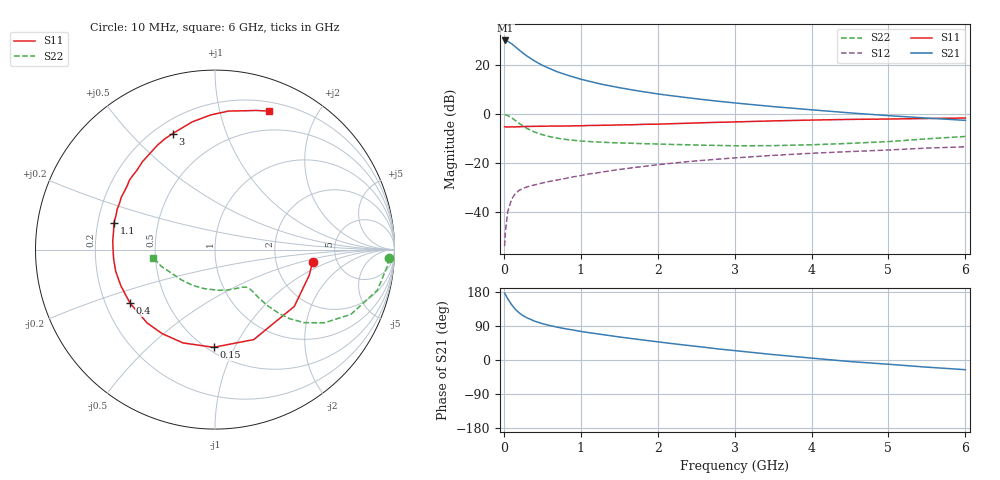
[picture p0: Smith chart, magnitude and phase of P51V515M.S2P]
! SIEMENS Small Signal Semiconductors
! BFP183
! Si NPN RF Bipolar Junction Transistor in SOT143
! VCE = 1.5 V  IC = 15 mA
! Common Emitter S-Parameters:  March  1996
# GHz  S  MA  R  50
!  f  S11  S21  S12  S22
! GHz  MAG  ANG  MAG  ANG  MAG  ANG  MAG  ANG
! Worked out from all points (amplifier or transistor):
!   36 points, 10 MHz to 6 GHz, reference 50 ohm
!   highest |S21| = 30.0 dB at 20 MHz (marker M1)
!   |S21| within 3 dB of that: start of sweep to 165.3 MHz
!   unconditionally stable (mu >= 1): 853.1 MHz to 5.693 GHz
!   at 250 MHz: K = 0.44, MSG = 27.6 dB, |S12| = -30.4 dB
!   at 1.4 GHz: K = 1.15, MAG = 14.9 dB, |S12| = -23.1 dB
!   at 6 GHz: K = 0.97, MSG = 5.4 dB, |S12| = -13.4 dB
!   S11 on the Smith chart (normalised r, x): 10 MHz: 3.29, -0.65; 150 MHz: 0.54, -0.83; 400 MHz: 0.30, -0.26; 1.1 GHz: 0.27, +0.12; 3 GHz: 0.27, +0.67; 6 GHz: 0.29, +1.42
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0.01  0.5485 -7.2  31.71 176.3  0.002 86.2  0.9715 -2.8
0.02  0.544 -15.3  31.73 172.9  0.0039 81.7  0.9635 -5.7
0.05  0.5436 -35.6  30.63 161.7  0.01 79.4  0.9328 -14.0
0.1  0.5458 -66.7  27.16 146.2  0.0182 64.0  0.8388 -25.5
0.15  0.5445 -90.8  23.52 133.7  0.0238 56.3  0.733 -33.8
0.2  0.5497 -108.9  20.23 124.3  0.0276 51.6  0.6425 -39.3
0.25  0.5531 -122.2  17.42 117.0  0.0302 47.8  0.5685 -42.7
0.3  0.5569 -132.7  15.29 111.4  0.0324 45.8  0.5082 -44.8
0.4  0.5596 -147.9  12.09 102.5  0.0357 45.1  0.4275 -46.9
0.5  0.5619 -159.0  9.865 96.0  0.039 44.4  0.3769 -47.6
0.6  0.5663 -167.5  8.407 90.8  0.0422 45.1  0.3436 -47.9
0.7  0.5671 -174.4  7.217 86.4  0.0451 46.5  0.3192 -48.0
0.9  0.572 174.9  5.718 79.1  0.052 48.1  0.2909 -48.6
1.1  0.5828 165.3  4.698 72.3  0.0593 48.8  0.2742 -50.1
1.5  0.5982 150.9  3.451 60.8  0.0736 49.3  0.2568 -54.8
1.8  0.6136 141.1  2.871 53.0  0.0843 48.3  0.2481 -60.1
2.2  0.6351 129.5  2.338 43.0  0.0993 45.9  0.2385 -68.5
3  0.6883 110.0  1.683 24.8  0.1268 40.1  0.2245 -90.1
3.5  0.723 100.1  1.416 14.3  0.1428 36.1  0.2257 -105.7
4.5  0.7756 84.4  1.053 -4.1  0.1708 27.4  0.2515 -137.7
5.5  0.8086 73.5  0.826 -18.9  0.2012 19.8  0.311 -162.0
6  0.8281 68.7  0.741 -25.6  0.2141 15.1  0.3476 -172.4
